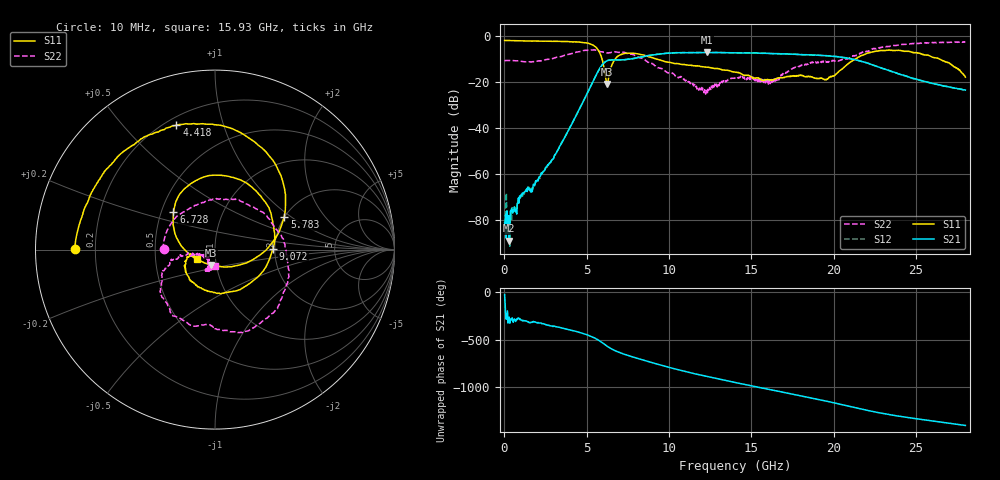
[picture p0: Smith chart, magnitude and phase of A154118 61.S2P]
!  2-Port S-parameters saved by WinCal
! VAR MeasName=S-Parameters (CALIBRATED_DATA) read from VNA (N5230A)
! VAR MeasDate=2015-9-10 14:39:49
! VAR NAME=A154118 61
! VAR FILENAME=A154118 61.S2P
! VAR DATE=2015-9-10 14:39:49
! VAR PHYS_PORTS=1,2
# Hz S DB R 50
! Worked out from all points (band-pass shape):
!   801 points, 10 MHz to 28 GHz, reference 50 ohm
!   highest |S21| = -7.35 dB at 12.29 GHz (marker M1); lowest = -88.8 dB at 289.9 MHz (marker M2)
!   |S21| within 3 dB of the highest: 7.407 GHz to 21.21 GHz (13.8 GHz wide, 96.4 % of centre)
!   lowest |S11| = -20.9 dB at 6.238 GHz (marker M3), VSWR 1.20, Z = 47 - j8.18 ohm
!   |S11| at or under -10 dB: 5.919 GHz to 6.742 GHz (823 MHz wide, 13 % of centre); 9.146 GHz to 21.35 GHz (12.2 GHz wide, 80 % of centre); 26.37 GHz to end of sweep
!   |S22| runs from -25.3 to -2.7 dB; largest |S21 - S12| = 0.0082
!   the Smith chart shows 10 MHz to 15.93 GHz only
!   S11 on the Smith chart (normalised r, x): 10 MHz: 0.12, +0.00; 4.418 GHz: 0.24, +0.71; 5.783 GHz: 1.99, +0.89; 6.728 GHz: 0.58, +0.27; 9.072 GHz: 1.95, +0.02; 15.93 GHz: 0.82, -0.08
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1e7  -2.15 179.7  -80.96 -25.5  -81.87 34.6  -10.94 179.7
2.899e8  -2.19 175.7  -88.79 96.6  -78.55 90.7  -10.79 166.7
2.564088e9  -2.46 145.3  -56.64 17.2  -57.03 15.8  -10.40 66.8
4.418425e9  -2.79 107.2  -33.71 -56.9  -33.73 -57.0  -7.17 -21.7
4.698325e9  -3.02 98.3  -29.81 -71.2  -29.81 -71.6  -6.75 -35.9
5.293112e9  -3.88 69.8  -21.17 -107.9  -21.20 -108.3  -6.27 -63.8
5.782938e9  -7.39 25.3  -14.34 -153.6  -14.34 -153.8  -6.88 -84.3
6.237775e9  -20.95 -105.6  -10.92 151.0  -10.91 150.9  -7.54 -94.0
6.7276e9  -10.13 137.9  -10.56 103.3  -10.57 103.3  -7.05 -106.8
7.70725e9  -7.66 77.4  -10.11 42.4  -10.13 42.2  -8.12 -140.1
9.071762e9  -9.82 1.0  -8.34 -27.3  -8.31 -27.2  -12.55 -165.5
9.351662e9  -10.40 -16.5  -8.09 -41.2  -8.05 -41.2  -13.90 -170.5
1.06462e10  -12.27 -88.1  -7.47 -101.3  -7.41 -101.5  -17.95 -170.2
1.229061e10  -13.73 -141.1  -7.35 -167.6  -7.30 -168.2  -24.13 -121.5
1.4005e10  -15.85 -164.0  -7.52 129.0  -7.51 128.4  -18.42 -112.1
1.592931e10  -19.15 -152.6  -7.73 61.0  -7.66 60.2  -20.59 -88.9
1.869332e10  -17.86 -139.0  -8.43 -35.6  -8.47 -36.2  -11.39 -82.7
1.9603e10  -18.70 -121.0  -8.78 -69.5  -8.73 -69.9  -11.29 -87.5
2.135238e10  -9.92 -105.8  -10.57 -138.1  -10.58 -138.7  -8.75 -81.0
2.334666e10  -6.38 -149.6  -15.10 152.3  -15.13 151.0  -4.76 -99.8
2.635559e10  -9.93 156.5  -21.26 74.6  -21.28 74.4  -3.09 -128.3
2.8e10  -18.03 131.6  -23.60 36.7  -23.67 36.2  -2.69 -141.1
